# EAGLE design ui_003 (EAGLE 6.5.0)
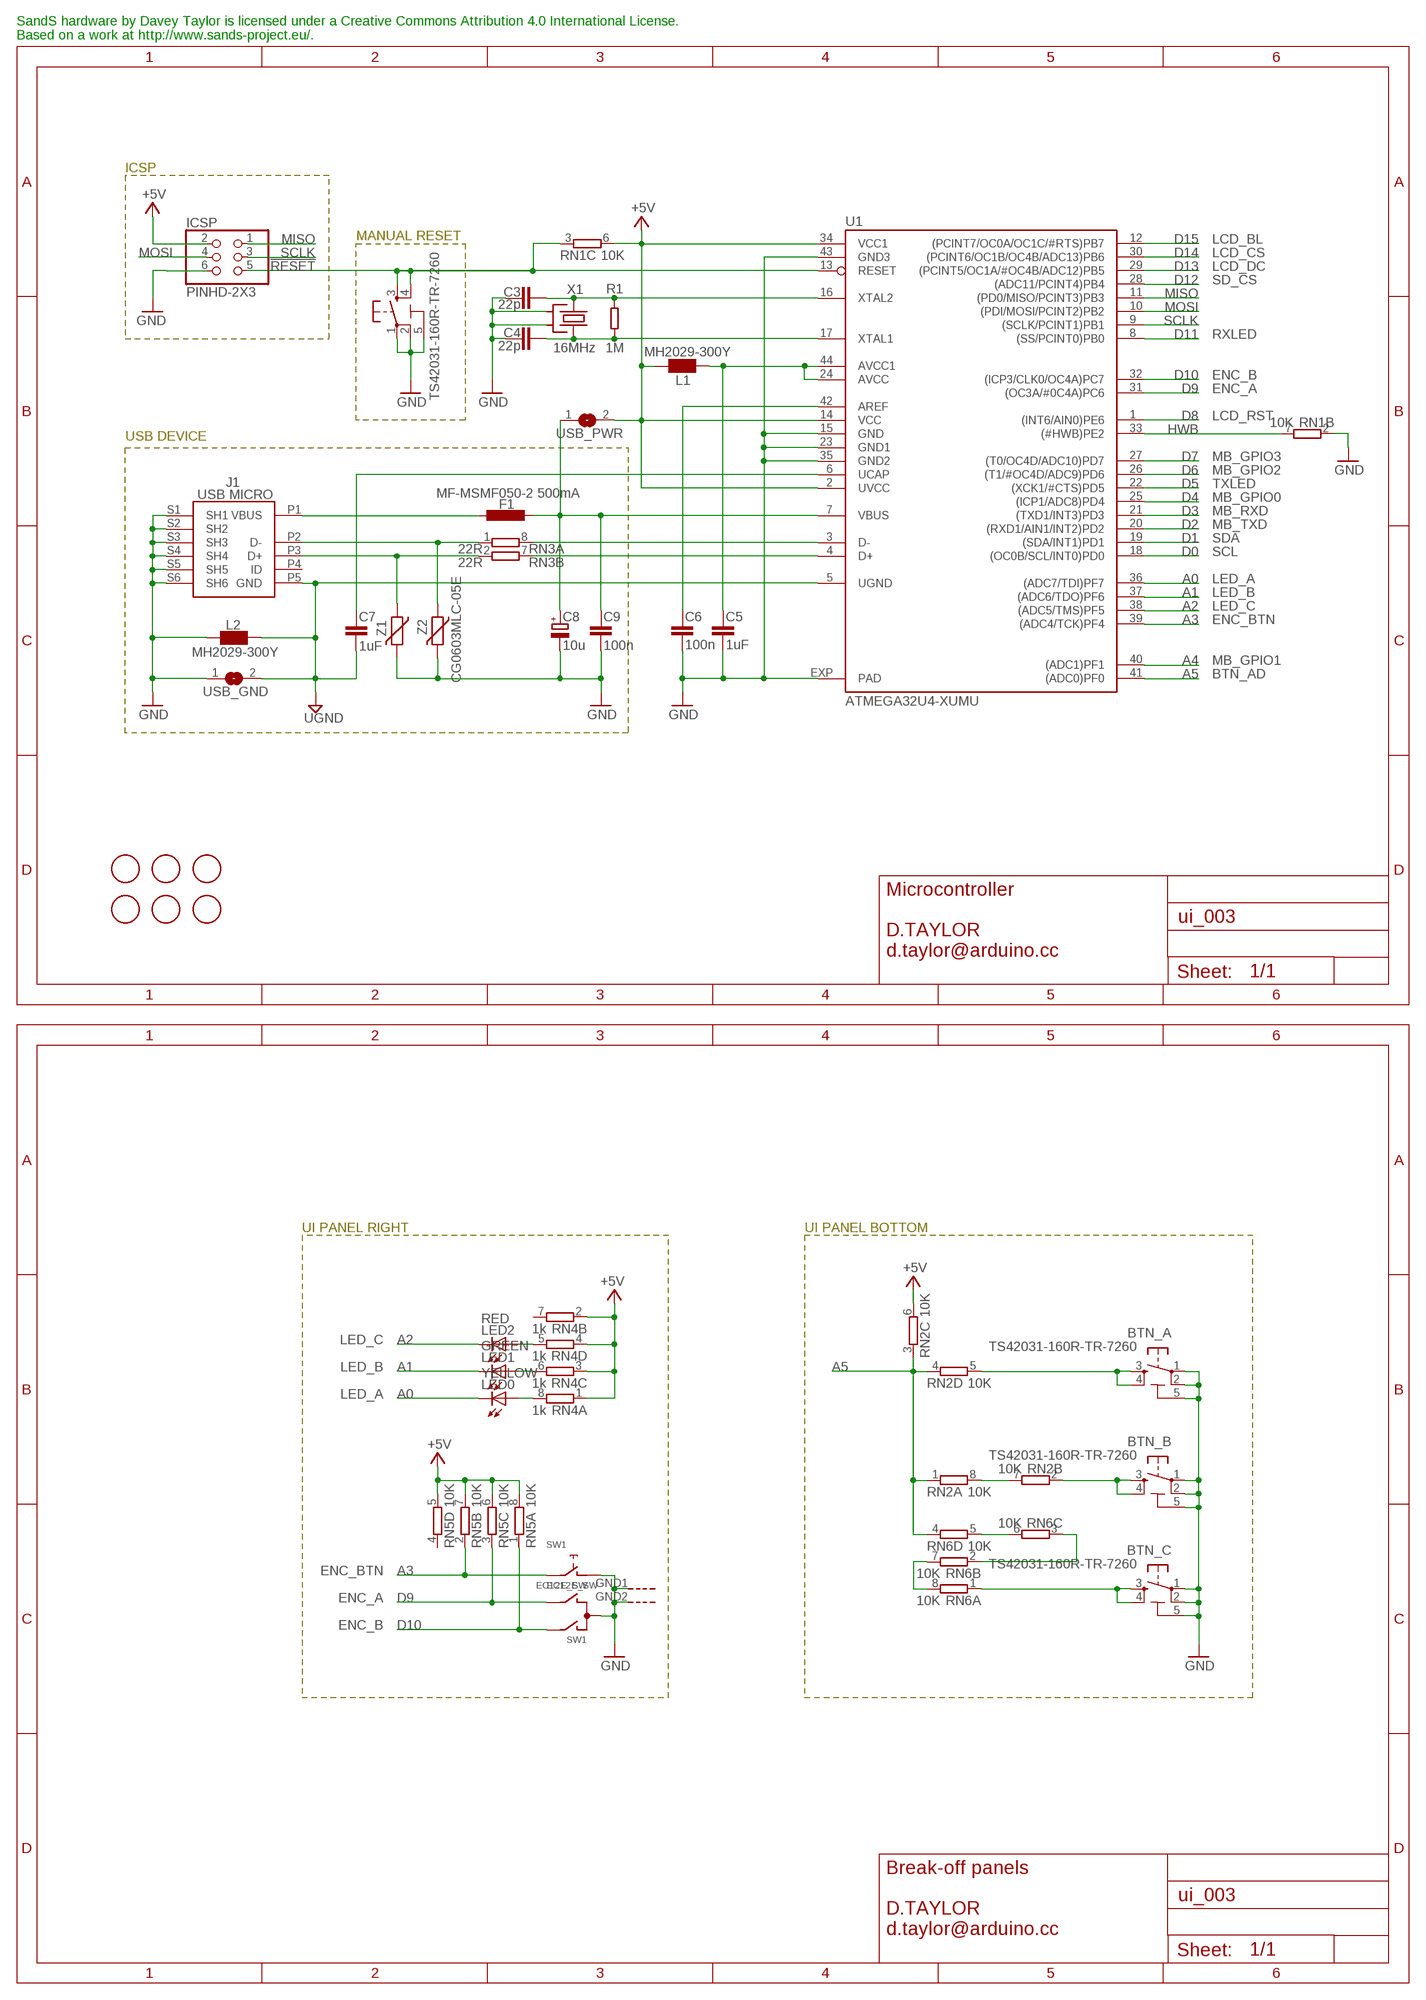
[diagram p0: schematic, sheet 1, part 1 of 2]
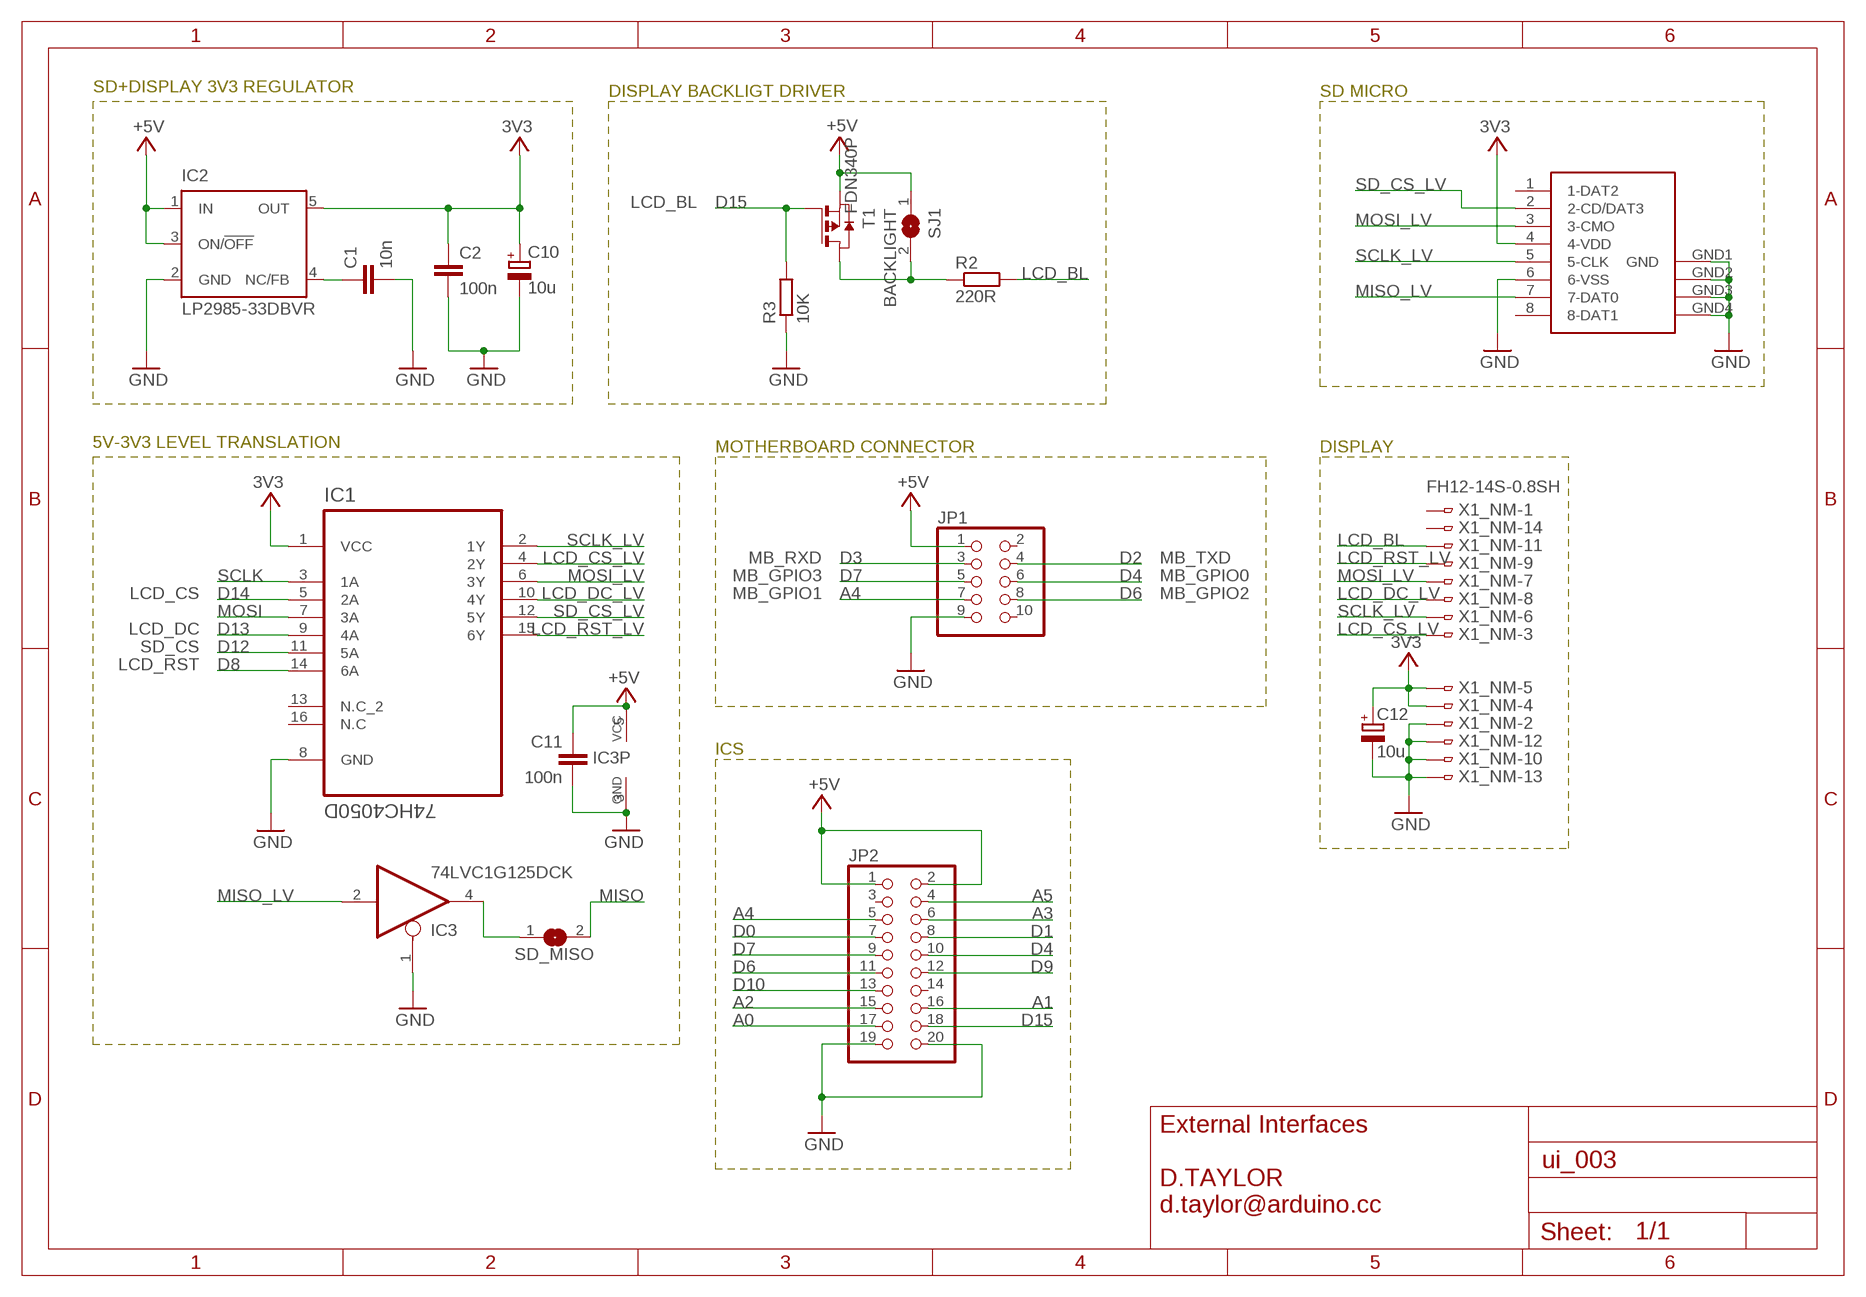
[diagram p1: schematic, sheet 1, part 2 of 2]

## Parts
BTN_A  TS42031-160R-TR-7260  TS42  [TS42]
BTN_B  TS42031-160R-TR-7260  TS42  [TS42]
BTN_C  TS42031-160R-TR-7260  TS42  [TS42]
C1  10n  C-EUC0603  [C0603-ROUND]
C2  100n  C-EUC0603  [C0603-ROUND]
C3  22p  C-EUC0603  [C0603-ROUND]
C4  22p  C-EUC0603  [C0603-ROUND]
C5  1uF  C-EUC0603  [C0603-ROUND]
C6  100n  C-EUC0603  [C0603-ROUND]
C7  1uF  C-EUC0603  [C0603-ROUND]
C8  10u  CPOL-EUSMCB  [SMC_B]
C9  100n  C-EUC0603  [C0603-ROUND]
C10  10u  CPOL-EUSMCB  [SMC_B]
C11  100n  C-EUC0603  [C0603-ROUND]
C12  10u  CPOL-EUSMCB  [SMC_B]
F1  MF-MSMF050-2 500mA  L-EUL1812  [L1812]
FID1  FIDUCIALMOUNT  [FIDUCIA-MOUNT]
FID2  FIDUCIALMOUNT  [FIDUCIA-MOUNT]
FID3  FIDUCIALMOUNT  [FIDUCIA-MOUNT]
FID4  FIDUCIALMOUNT  [FIDUCIA-MOUNT]
FID5  FIDUCIALMOUNT  [FIDUCIA-MOUNT]
FID6  FIDUCIALMOUNT  [FIDUCIA-MOUNT]
IC1  74HC4050D  [SOIC127P600X175-16N]
IC2  LP2985-33DBVR  LP2985-XXDBVR33  [SOT23-DBV]
IC3  74LVC1G125DCK  [SC70-5]
ICSP  PINHD-2X3  [2X03]
J1  USB MICRO  MYCON2_USB-MINI-B  [CON2_USB_MICRO_B_AT]
JP1  PINHD-2X5  [2X05]
JP2  PINHD-2X10  [2X10]
L1  MH2029-300Y  WE-CBF_0805  [0805]
L2  MH2029-300Y  WE-CBF_0805  [0805]
LED0  YELLOW  LEDCHIPLED_0805  [CHIPLED_0805]
LED1  GREEN  LEDCHIPLED_0805  [CHIPLED_0805]
LED2  RED  LEDCHIPLED_0805  [CHIPLED_0805]
R1  1M  R-EU_0603-RND  [R0603-ROUND]
R2  220R  R-EU_0603-RND  [R0603-ROUND]
R3  10K  R-EU_0603-RND  [R0603-ROUND]
RESET  TS42031-160R-TR-7260  TS42  [TS42]
RN1  10K  4R-NCAY16  [CAY16]
RN2  10K  4R-NCAY16  [CAY16]
RN3  22R  4R-NCAY16  [CAY16]
RN4  1k  4R-NCAY16  [CAY16]
RN5  10K  4R-NCAY16  [CAY16]
RN6  10K  4R-NCAY16  [CAY16]
SD_MISO  SJ-NO  [SJ]
SJ1  BACKLIGHT  SJ-NO  [SJ]
SW1  EC12E_SW  [ALPS_EC12E_SW]
T1  FDN340P  [SOT-23]
U1  ATMEGA32U4-XUMU  [QFN44ML7X7]
U2  SDCARD-15TW-8821  [SDCARD-15TW-8821]
USB_GND  SJ-NO  [SJ]
USB_PWR  SJ-NO  [SJ]
X1  16MHz  CRYSTAL2-KX7  [XTAL-3.2-2.5]
X1_NM  FH12-14S-0.8SH  [FH12-14S-0.5SH]
Z1  CG0603MLC-05E  VARISTORCN0603  [CT/CN0603]
Z2  CG0603MLC-05E  VARISTORCN0603  [CT/CN0603]

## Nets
3V3: C2.1 C10.+ C12.+ IC1.1(VCC) IC2.5(OUT) U2.4(4-VDD) X1_NM.4 X1_NM.5
!RESET!: ICSP.5 RESET.3 RESET.4 RN1.3 U1.13(RESET)
+5V [usbvcc]: C11.1 IC2.1(IN) IC2.3(ON/!OFF) IC3.5(VCC) ICSP.2 JP1.1 JP2.1 JP2.2 L1.1 RN1.6 RN2.6 RN4.1 RN4.2 RN4.3 RN4.4 RN5.5 RN5.6 RN5.7 RN5.8 SJ1.1 T1.2(S) U1.2(UVCC) U1.14(VCC) U1.34(VCC1) USB_PWR.2
A0: JP2.17 LED0.C U1.36((ADC7/TDI)PF7)
A1: JP2.16 LED1.C U1.37((ADC6/TDO)PF6)
A2: JP2.15 LED2.C U1.38((ADC5/TMS)PF5)
A3: JP2.6 RN5.2 SW1.E U1.39((ADC4/TCK)PF4)
A4: JP1.7 JP2.5 U1.40((ADC1)PF1)
A5: JP2.4 RN2.1 RN2.3 RN2.4 RN6.4 U1.41((ADC0)PF0)
AREF [aref]: C6.1 U1.42(AREF)
AVCC: C5.1 L1.2 U1.24(AVCC) U1.44(AVCC1)
D0: JP2.7 U1.18((OC0B/SCL/INT0)PD0)
D1: JP2.8 U1.19((SDA/INT1)PD1)
D2: JP1.4 U1.20((RXD1/AIN1/INT2)PD2)
D3: JP1.3 U1.21((TXD1/INT3)PD3)
D4: JP1.6 JP2.10 U1.25((ICP1/ADC8)PD4)
D5: U1.22((XCK1/#CTS)PD5)
D6: JP1.8 JP2.11 U1.26((T1/#OC4D/ADC9)PD6)
D7: JP1.5 JP2.9 U1.27((T0/OC4D/ADC10)PD7)
D8: IC1.14(6A) U1.1((INT6/AIN0)PE6)
D9: JP2.12 RN5.3 SW1.B U1.31((OC3A/#0C4A)PC6)
D10: JP2.13 RN5.1 SW1.A U1.32((ICP3/CLK0/OC4A)PC7)
D11: U1.8((SS/PCINT0)PB0)
D12: IC1.11(5A) U1.28((ADC11/PCINT4)PB4)
D13: IC1.9(4A) U1.29((PCINT5/OC1A/#OC4B/ADC12)PB5)
D14: IC1.5(2A) U1.30((PCINT6/OC1B/OC4B/ADC13)PB6)
D15: JP2.18 R3.2 T1.1(G) U1.12((PCINT7/OC0A/OC1C/#RTS)PB7)
D+: J1.P3(D+) RN3.2 Z1.1
D-: J1.P2(D-) RN3.1 Z2.1
GND [gnd]: BTN_A.1 BTN_A.2 BTN_A.5(5-GND) BTN_B.1 BTN_B.2 BTN_B.5(5-GND) BTN_C.1 BTN_C.2 BTN_C.5(5-GND) C1.2 C2.2 C3.1 C4.2 C5.2 C6.2 C8.- C9.2 C10.- C11.2 C12.- IC1.8(GND) IC2.2(GND) IC3.1(OE) IC3.3(GND) ICSP.6 J1.S1(SH1) J1.S2(SH2) J1.S3(SH3) J1.S4(SH4) J1.S5(SH5) J1.S6(SH6) JP1.9 JP2.19 JP2.20 L2.2 R3.1 RESET.1 RESET.2 RESET.5(5-GND) RN1.2 SW1.C SW1.D SW1.GND1(G) SW1.GND2(G) U1.15(GND) U1.23(GND1) U1.35(GND2) U1.43(GND3) U1.EXP(PAD) U2.6(6-VSS) U2.GND1(GND) U2.GND2(GND1) U2.GND3(GND2) U2.GND4(GND3) USB_GND.1 X1.2(SH1) X1.4(SH2) X1_NM.2 X1_NM.10 X1_NM.12 X1_NM.13 Z1.2 Z2.2
HWB: RN1.7 U1.33((#HWB)PE2)
LCD_BL: R2.2 X1_NM.11
LCD_CS_LV: IC1.4(2Y) X1_NM.3
LCD_DC_LV: IC1.10(4Y) X1_NM.8
LCD_RST_LV: IC1.15(6Y) X1_NM.9
MISO: ICSP.1 SD_MISO.2 U1.11((PD0/MISO/PCINT3)PB3)
MISO_LV: IC3.2(I) U2.7(7-DAT0)
MOSI: IC1.7(3A) ICSP.4 U1.10((PDI/MOSI/PCINT2)PB2)
MOSI_LV: IC1.6(3Y) U2.3(3-CMO) X1_NM.7
N$2: R2.1 SJ1.2 T1.3(D)
N$3: C1.1 IC2.4(NC/FB)
N$4: LED0.A RN4.8
N$5: LED2.A RN4.5
N$6: LED1.A RN4.6
N$7: BTN_A.3 BTN_A.4 RN2.5
N$8: IC3.4(O) SD_MISO.1
N$9: RN2.7 RN2.8
N$10: RN6.5 RN6.6
N$11: BTN_B.3 BTN_B.4 RN2.2
N$12: BTN_C.3 BTN_C.4 RN6.1
N$13: RN6.2 RN6.3
N$14: RN6.7 RN6.8
SCLK: IC1.3(1A) ICSP.3 U1.9((SCLK/PCINT1)PB1)
SCLK_LV: IC1.2(1Y) U2.5(5-CLK) X1_NM.6
SD_CS_LV: IC1.12(5Y) U2.2(2-CD/DAT3)
UCAP: C7.1 U1.6(UCAP)
UGND [gnd]: C7.2 J1.P5(GND) L2.1 U1.5(UGND) USB_GND.2
USB_D+: RN3.7 U1.4(D+)
USB_D-: RN3.8 U1.3(D-)
USB_VCC: C8.+ C9.1 F1.1 U1.7(VBUS) USB_PWR.1
XTAL1: C4.1 R1.1 U1.17(XTAL1) X1.3(X2)
XTAL2: C3.2 R1.2 U1.16(XTAL2) X1.1(X1)
XUSB [usbvcc]: F1.2 J1.P1(VBUS)
Unconnected: IC1.13(N.C_2) IC1.16(N.C) J1.P4(ID) JP1.2 JP1.10 JP2.3 JP2.14 RN1.1 RN1.4 RN1.5 RN1.8 RN3.3 RN3.4 RN3.5 RN3.6 RN4.7 RN5.4 U2.1(1-DAT2) U2.8(8-DAT1) X1_NM.1 X1_NM.14

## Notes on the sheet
- SandS hardware by Davey Taylor is licensed under a Creative Commons Attribution 4.0 International License.
  Based on a work at http://www.sands-project.eu/.
- ICSP
- MANUAL RESET | LCD_BL
- LCD_CS
- LCD_DC
- SD_CS
- RXLED
- ENC_B
- ENC_A
- LCD_RST
- USB DEVICE
- MB_GPIO3
- MB_GPIO2
- TXLED
- MB_GPIO0
- MB_RXD
- MB_TXD
- SDA
- SCL
- LED_A
- LED_B
- LED_C
- ENC_BTN
- MB_GPIO1
- BTN_AD
- Microcontroller
  
  D.TAYLOR
  d.taylor@arduino.cc
- UI PANEL RIGHT | UI PANEL BOTTOM
- LED_C
- LED_B
- LED_A
- ENC_BTN
- ENC_A
- ENC_B
- Break-off panels
  
  D.TAYLOR
  d.taylor@arduino.cc
- SD+DISPLAY 3V3 REGULATOR | DISPLAY BACKLIGT DRIVER | SD MICRO
- LCD_BL
- 5V-3V3 LEVEL TRANSLATION | MOTHERBOARD CONNECTOR | DISPLAY
- MB_RXD | MB_TXD
- MB_GPIO3 | MB_GPIO0
- LCD_CS | MB_GPIO1 | MB_GPIO2
- LCD_DC
- SD_CS
- LCD_RST
- ICS
- External Interfaces
  
  D.TAYLOR
  d.taylor@arduino.cc

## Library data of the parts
BTN_A BTN_B BTN_C RESET = SmartPrj:TS42: TS42 Dongnan Electronics Tact switch VDC 12V - 50mA
C1-C7 C9 C11 = SmartPrj:C-EU: CAPACITOR, European symbol
C8 C12 = rcl:CPOL-EU: POLARIZED CAPACITOR, European symbol
C10 = SmartPrj:CPOL-EU: POLARIZED CAPACITOR, European symbol
F1 = rcl:L-EU: INDUCTOR, European symbol
FID1-FID6 = SmartPrj:FIDUCIALMOUNT
IC1 = SmartPrj:74HC4050D: Hex high-to-low level shifter; MPN: 74HC4050D; OC_FARNELL: 1085272; OC_NEWARK: -; PACKAGE: SOIC-16; SUPPLIER: NXP
IC2 = SmartPrj:LP2985-XXDBVR: ULTRALOW-POWER 50-mA LOW-DROPOUT LINEAR REGULATORS 50-mA Low-Dropout Regulator Source: http://focus.ti.com/lit/ds/symlink/tps77001.pdf
IC3 = 74xx-little-us:74*1G125: Single Bus Buffer Gate with 3-State Output
ICSP = SmartPrj:PINHD-2X3: PIN HEADER
J1 = d_taylor:MYCON2_USB-MINI-B
JP1 = pinhead:PINHD-2X5: PIN HEADER
JP2 = pinhead:PINHD-2X10: PIN HEADER
L1 L2 = wuerth-elektronik:WE-CBF: SMD EMI Suppression Ferrite Beads
LED0 LED1 LED2 = led:LED: LED
R1 = d_taylor:R-EU_: RESISTOR, European symbol
R2 R3 = SmartPrj:R-EU_: RESISTOR, European symbol
RN1-RN6 = resistor-dil:4R-N: Array Chip Resistor Source: RS Component / Phycomp; OC_FARNELL: unknown; OC_NEWARK: unknown
SD_MISO SJ1 USB_GND USB_PWR = d_taylor:SJ?-NO: SMD solder JUMPER
SW1 = switch-alps:EC12E_SW: ALPS rotary Encoder EC12E series with switch; MPN: EC12E2424407; OC_FARNELL: 1520813; OC_NEWARK: 74M1068
T1 = d_taylor:FDN340
U1 = d_taylor:ATMEGA32U4-XU
U2 = st-mod v1.4:SDCARD-15TW-8821: SD Card SDCARD 15TW 8821
X1 = d_taylor:CRYSTAL2: KX7 SMD crystal
X1_NM = con-hirose:FH12-14S-0.8S: 0.5mm Pitch Connectors For FPC/FFC Source: Data sheet; MPN: MC34827; OC_FARNELL: 1324544; OC_NEWARK: 41P0493
Z1 Z2 = varistor:VARISTOR: VARISTOR

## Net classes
0 default: width 0.203 mm, drill 0.406 mm, clearance 0.203 mm
2 gnd: width 0.203 mm, drill 0.406 mm, clearance 0.203 mm
3 usbvcc: width 0.203 mm, drill 0.406 mm, clearance 0.203 mm
4 aref: width 0.203 mm, drill 0.406 mm, clearance 0.203 mm

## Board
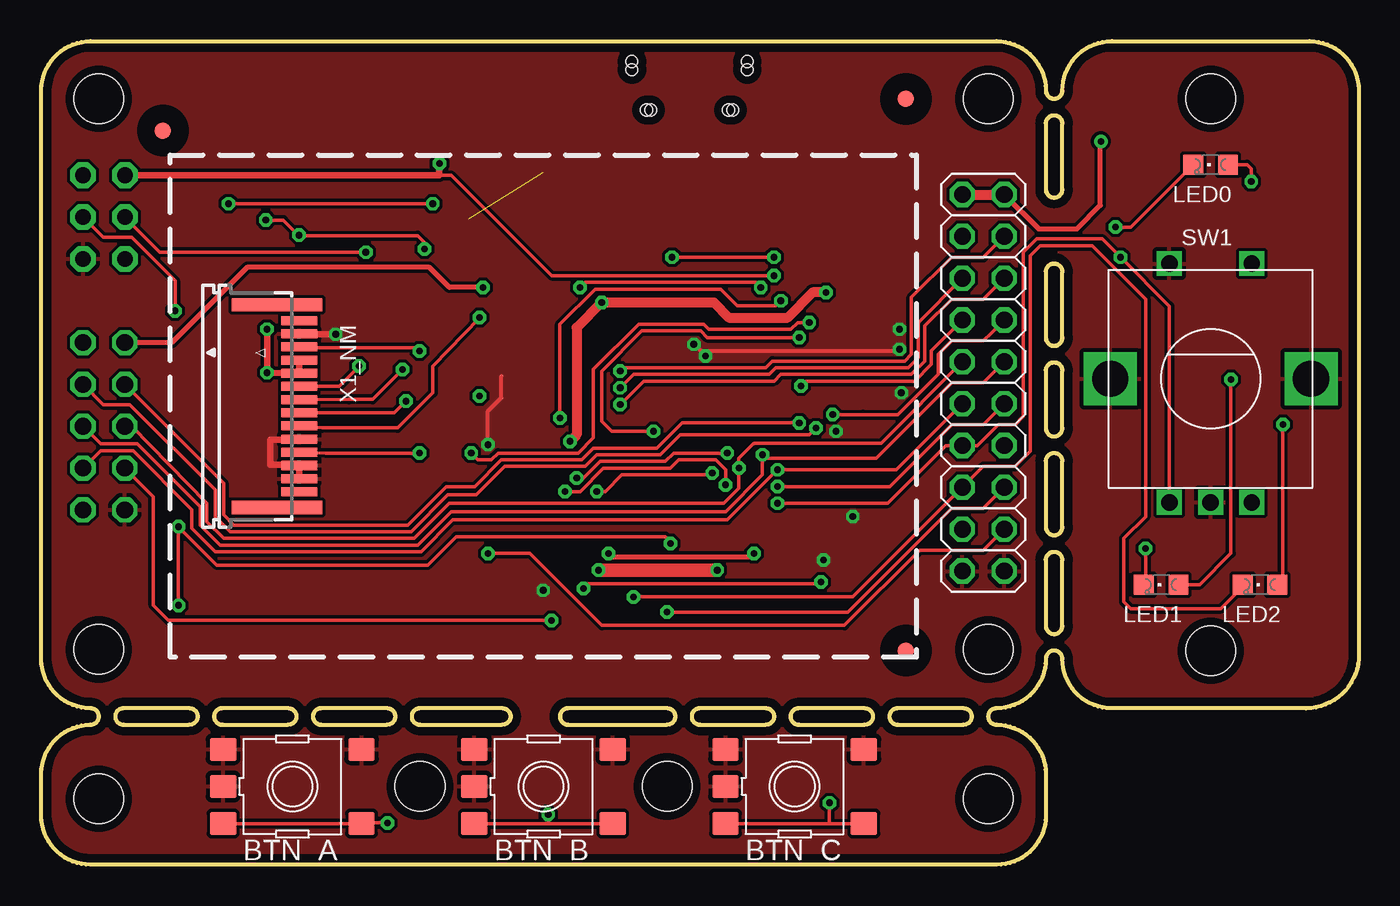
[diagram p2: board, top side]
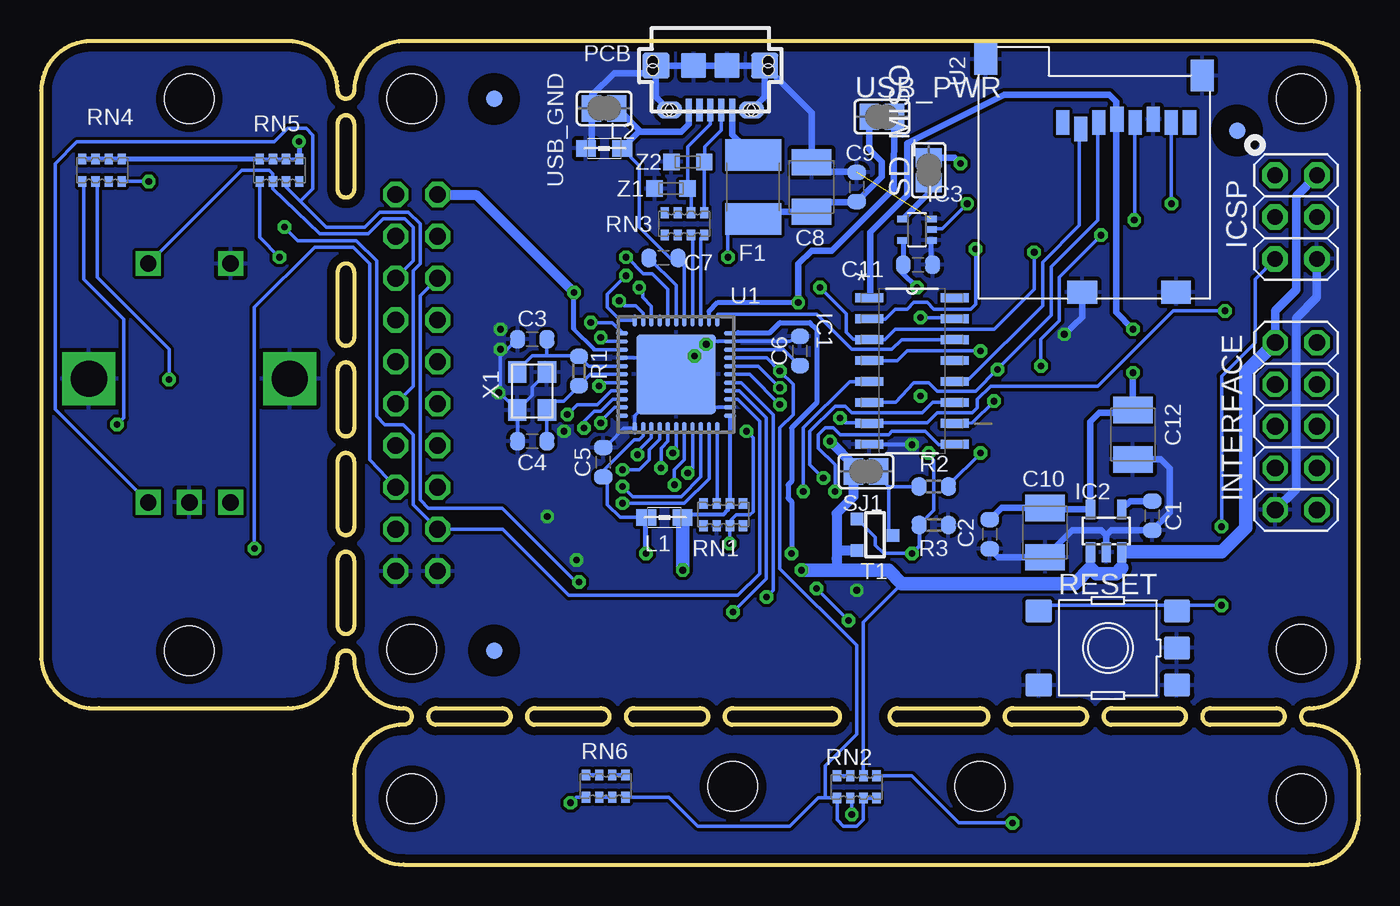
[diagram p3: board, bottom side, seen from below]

Size 80 x 50 mm. Coordinates in mm from the lower left corner, seen from the top.
Outline: 76 segments
Copper layers (1*16): Top 0.035mm / dielectric 1.5mm / Bottom 0.035mm
Design rules "default *": minimum track width 8mil, minimum drill 16mil, track to track 8mil, track to pad 8mil, pad to pad 8mil, via to via 8mil, smd to smd 8mil, copper to edge 20mil, drill to drill 8mil, minimum pad ring 10mil, minimum via ring 8mil, stop-mask expansion 4mil, vias tented up to drill 0mil, thermal gap 10mil
Holes 3 mm at 3.5,46.5 3.5,4 57.5,4 57.5,46.5 3.5,13.07 57.5,13.07 71,46.5 71,13 38,4.75 23,4.75

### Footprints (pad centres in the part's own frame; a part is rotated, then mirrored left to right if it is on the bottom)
TS42 = smd 1.6 x 1.4: 1 -4.2,2.25; 2 4.2,2.25; 3 -4.2,-2.25; 4 4.2,-2.25; 5 -4.2,0
C0603-ROUND = smd 0.898 x 1.1: 1 -0.889,0; 2 0.889,0
SMC_B = smd 1.6 x 2.4: + -1.5,0; - 1.5,0
L1812 = smd 1.9 x 3.4: 1 -1.95,0; 2 1.95,0
FIDUCIA-MOUNT = smd 1.016 x 1.016: P$1 0,0
SOIC127P600X175-16N = smd 1.702 x 0.533: 1 -2.591,4.445; 2 -2.591,3.175; 3 -2.591,1.905; 4 -2.591,0.635; 5 -2.591,-0.635; 6 -2.591,-1.905; 7 -2.591,-3.175; 8 -2.591,-4.445; 9 2.591,-4.445; 10 2.591,-3.175; 11 2.591,-1.905; 12 2.591,-0.635; 13 2.591,0.635; 14 2.591,1.905; 15 2.591,3.175; 16 2.591,4.445
SOT23-DBV = smd 0.55 x 1.2: 1 -0.95,-1.3; 2 0,-1.3; 3 0.95,-1.3; 4 0.95,1.3; 5 -0.95,1.3
SC70-5 = smd 0.4 x 0.7: 1 -0.65,-0.85; 2 0,-0.85; 3 0.65,-0.85; 4 0.65,0.85; 5 -0.65,0.85
2X03 = drill 0.95 pad 1.55 octagon: 1 -2.54,-1.27; 2 -2.54,1.27; 3 0,-1.27; 4 0,1.27; 5 2.54,-1.27; 6 2.54,1.27
CON2_USB_MICRO_B_AT = smd 0.406 x 1.346: P1 -1.321,2.692; P2 -0.66,2.692; P3 0,2.692; P4 0.66,2.692; P5 1.321,2.692 | smd 1.651 x 1.549: S1 -3.302,0; S2 3.302,0 | smd 1.524 x 1.016: S3 -2.489,2.692; S4 2.489,2.692 | smd 1.524 x 1.524: S5 -1.016,0; S6 1.016,0 | hole 0.7: -3.505,0.254; -3.505,-0.254; 3.505,0.254; 3.505,-0.254; -2.616,2.692; -2.362,2.692; 2.362,2.692; 2.616,2.692
2X05 = drill 1.016 octagon: 1 -5.08,-1.27; 2 -5.08,1.27; 3 -2.54,-1.27; 4 -2.54,1.27; 5 0,-1.27; 6 0,1.27; 7 2.54,-1.27; 8 2.54,1.27; 9 5.08,-1.27; 10 5.08,1.27
2X10 = drill 1.016 octagon: 1 -11.43,-1.27; 2 -11.43,1.27; 3 -8.89,-1.27; 4 -8.89,1.27; 5 -6.35,-1.27; 6 -6.35,1.27; 7 -3.81,-1.27; 8 -3.81,1.27; 9 -1.27,-1.27; 10 -1.27,1.27; 11 1.27,-1.27; 12 1.27,1.27; 13 3.81,-1.27; 14 3.81,1.27; 15 6.35,-1.27; 16 6.35,1.27; 17 8.89,-1.27; 18 8.89,1.27; 19 11.43,-1.27; 20 11.43,1.27
0805 = smd 1.2 x 1: 1 -1.1,0; 2 1.1,0
CHIPLED_0805 = smd 1.2 x 1.2: A 0,-1.05; C 0,1.05
R0603-ROUND = smd 0.898 x 1.1: 1 -0.889,0; 2 0.889,0
CAY16 = smd 0.5 x 0.65: 1 -1.2,-0.675; 2 -0.4,-0.675; 3 0.4,-0.675; 4 1.2,-0.675; 5 1.2,0.675; 6 0.4,0.675; 7 -0.4,0.675; 8 -1.2,0.675
SJ = smd 1.168 x 1.6: 1 -0.762,0; 2 0.762,0
ALPS_EC12E_SW = drill 1 square: A -2.5,-7.5; B 2.5,-7.5; C 0,-7.5; D -2.5,7; E 2.5,7 | drill 2.2 square: GND1 -6.1,0; GND2 6.1,0
SOT-23 = smd 0.762 x 0.762: 1 -0.979,-1.101; 2 0.94,-1.101; 3 0.025,1.067
QFN44ML7X7 = smd 0.75 x 0.275: 1 -3.275,2.5; 2 -3.275,2; 3 -3.275,1.5; 4 -3.275,1; 5 -3.275,0.5; 6 -3.275,0; 7 -3.275,-0.5; 8 -3.275,-1; 9 -3.275,-1.5; 10 -3.275,-2; 11 -3.275,-2.5; 23 3.275,-2.5; 24 3.275,-2; 25 3.275,-1.5; 26 3.275,-1; 27 3.275,-0.5; 28 3.275,0; 29 3.275,0.5; 30 3.275,1; 31 3.275,1.5; 32 3.275,2; 33 3.275,2.5 | smd 0.275 x 0.75: 12 -2.5,-3.275; 13 -2,-3.275; 14 -1.5,-3.275; 15 -1,-3.275; 16 -0.5,-3.275; 17 0,-3.275; 18 0.5,-3.275; 19 1,-3.275; 20 1.5,-3.275; 21 2,-3.275; 22 2.5,-3.275; 34 2.5,3.275; 35 2,3.275; 36 1.5,3.275; 37 1,3.275; 38 0.5,3.275; 39 0,3.275; 40 -0.5,3.275; 41 -1,3.275; 42 -1.5,3.275; 43 -2,3.275; 44 -2.5,3.275 | smd 4.826 x 4.826: EXP 0,0
SDCARD-15TW-8821 = smd 0.8 x 1.5: 1 0,0; 2 1.1,-0.4; 3 2.2,0; 4 3.3,0.2; 5 4.4,0; 6 5.5,0.2; 7 6.6,0; 8 7.7,0 | smd 1.4 x 1.9: GND1 -4.66,3.85; GND2 8.49,2.85 | smd 1.8 x 1.4: GND3 1.19,-10.3; GND4 6.89,-10.3
XTAL-3.2-2.5 = smd 1.3 x 1.1: 1 -1.15,-0.9; 2 1.15,-0.9; 3 1.15,0.9; 4 -1.15,0.9
FH12-14S-0.5SH = smd 0.55 x 2.2: 1 -5.2,3.25; 2 -4.4,3.25; 3 -3.6,3.25; 4 -2.8,3.25; 5 -2,3.25; 6 -1.2,3.25; 7 -0.4,3.25; 8 0.4,3.25; 9 1.2,3.25; 10 2,3.25; 11 2.8,3.25; 12 3.6,3.25; 13 4.4,3.25; 14 5.2,3.25 | smd 0.8 x 5.5: P1 -6.15,1.9; P2 6.15,1.9
CT/CN0603 = smd 1 x 1: 1 -1,0; 2 1,0

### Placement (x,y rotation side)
BTN_A  15.25,4.75 0 top
BTN_B  30.5,4.75 0 top
BTN_C  45.75,4.75 0 top
C1  12.55,21.18 270 bottom
C2  22.4,20.07 270 bottom
C3  50.19,31.9 0 bottom
C4  50.19,25.7 180 bottom
C5  45.87,24.43 90 bottom
C6  33.93,31.19 90 bottom
C7  42.21,36.83 0 bottom
C8  33.22,41.15 90 bottom
C9  30.48,41.15 90 bottom
C10  19.05,20.17 270 bottom
C11  26.77,36.42 0 bottom
C12  13.72,26.11 270 bottom
F1  36.78,41.15 90 bottom
FID1  52.5,13 0 bottom
FID2  7.38,44.57 0 bottom
FID3  52.5,46.5 0 bottom
FID4  7.38,44.57 0 top
FID5  52.5,46.5 0 top
FID6  52.5,13 0 top
IC1  27.13,29.97 0 bottom
IC2  15.34,20.27 0 bottom
IC3  26.82,38.56 90 bottom
ICSP  3.81,39.32 270 bottom
J1  39.37,48.51 180 bottom
JP1  3.81,26.62 270 bottom
JP2  57.2,29.26 270 top
L1  42.16,21.08 180 bottom
L2  45.82,43.48 180 bottom
LED0  71,42.5 90 top
LED1  68,17 90 top
LED2  74,17 90 top
R1  47.35,29.97 90 bottom
R2  25.81,22.96 0 bottom
R3  25.81,20.62 180 bottom
RESET  15.24,13.16 180 bottom
RN1  38.58,21.26 0 bottom
RN2  30.48,4.72 0 bottom
RN3  40.94,38.91 180 bottom
RN4  76.3,42.16 180 bottom
RN5  65.53,42.16 0 bottom
RN6  45.72,4.78 0 bottom
SD_MISO  26.11,42.16 90 bottom
SJ1  29.92,23.88 0 bottom
SW1  71,29.5 0 top
T1  29.36,20.02 270 bottom
U1  41.45,29.77 270 bottom
U2  17.98,45.06 0 bottom
USB_GND  45.82,45.92 0 bottom
USB_PWR  28.96,45.42 0 bottom
X1  50.19,28.75 270 bottom
X1_NM  12.42,27.84 270 top
Z1  41.76,41.05 180 bottom
Z2  40.74,42.67 180 bottom

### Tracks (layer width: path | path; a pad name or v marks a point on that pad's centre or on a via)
3V3  (via drill 0.41)
  Top 0.406: v13.72,32.51 v13.72,29.87 15.61,29.84 X1_NM.5 X1_NM.4
  Bottom 0.203: 14.73,44.91 U2.4 14.73,45.31
  Bottom 0.406: v13.72,32.51 14.73,33.53 14.73,44.91 | IC1.1 29.69,34.42 29.67,34.44 29.67,38.41 27.43,40.64 27.43,43.79 21.54,46.74 15.14,46.74 14.73,46.33 14.73,45.31 | C2.1 21.69,21.67 C10.+ 18.95,21.57 IC2.5 16.29,26.89 15.75,27.43 13.89,27.43 C12.+ v13.72,29.87
!RESET!  (via drill 0.41)
  Top 0.203: v8.33,15.75 v8.33,20.52 10.67,18.19 23.47,18.19 25.2,19.91 37.9,19.91 v38.2,19.51 | v37.19,26.31 34.65,26.31 34.04,26.92 34.04,29.97 36.47,32.41 40.03,32.41 40.44,32 v46.02,32
  Bottom 0.203: ICSP.5 6.3,35.56 6.3,31.7 8.33,29.67 v8.33,20.52 | RESET.3 10.69,15.75 v8.33,15.75 18.93,15.75 RESET.4 | v38.2,19.51 38.2,20.42 RN1.3 38.1,20.77 38.1,20.93 37.8,21.23 36.98,21.23 36.78,21.44 36.78,25.91 v37.19,26.31 | v46.02,32 45.79,31.77 U1.13
+5V  (via drill 0.41)
  Top 0.305: v26.82,35.05 24.79,35.05 23.57,36.27 12.5,36.27 7.92,31.7 JP1.1 | JP2.2 60.55,38.61 62.89,38.61 64.31,40.03 64.31,43.89 v64.34,43.92
  Top 0.61: v32.11,25.7 32.51,26.11 32.51,32.61 v34.04,34.14 40.84,34.14 41.76,33.22 45.31,33.22 46.84,34.75 v47.65,34.75 | JP2.1 JP2.2
  Top 0.813: v41.05,17.88 v33.83,17.88
  Bottom 0.203: 41.05,21.26 L1.1 | 27.67,36.44 C11.1 27.74,36.6 | 27.74,17.07 30.07,14.73 30.07,5.49 RN2.6 | 38.28,21.66 38.28,21.86 RN1.6 38.18,22.04 | U1.14 46.41,31.27 46.43,31.29 | RN5.8 RN5.7 RN5.6 RN5.5
  Bottom 0.254: 41.05,21.26 38.58,21.26 38.3,21.54 38.28,21.66 | U1.2 39.45,33.6 | 38.18,22.04 U1.34 | 46.43,31.29 47.65,32.51 | 30.73,18.03 30.89,17.88
  Bottom 0.305: IC3.5 27.67,36.44 | 27.74,36.6 27.74,35.97 v26.82,35.05 | 3.86,40.54 3.81,40.59 | 39.45,33.6 38.91,34.14 v34.04,34.14 | 30.68,24.28 SJ1.1 | 47.65,32.51 v47.65,34.75 | L1.1 41.06,20.85 41.05,20.83 | RN4.4 RN4.3 RN4.2 RN4.1 RN5.8 | v64.34,43.92 RN5.5
  Bottom 0.406: IC2.3 14.39,18.02 | IC2.1 16.29,18.02 | 17.24,17.07 17.27,17.07 | USB_PWR.2 28.25,41.05 32,37.29 33.22,37.29 34.04,36.47 v34.04,34.14
  Bottom 0.508: IC2.3 14.36,18.97 14.22,19 | JP1.1 5.08,33.63 3.81,34.9 3.81,40.59 ICSP.2
  Bottom 0.61: v32.11,25.7 30.68,24.28 | v47.65,34.75 53.54,40.64 55.88,40.64 JP2.1 | SJ1.1 30.68,22.35 31.7,21.34 31.7,18.59 | 31.7,18.59 31.7,17.88 | T1.2 31.67,19.07 31.7,18.59
  Bottom 0.813: 14.39,18.02 14.73,17.68 15.95,17.68 16.29,18.02 17.24,17.07 | 14.22,19 8.33,19 6.86,20.47 6.86,29.92 JP1.1 | 17.27,17.07 27.74,17.07 28.55,17.88 30.89,17.88 31.7,17.88 v33.83,17.88 | 41.05,20.83 v41.05,17.88
A0  (via drill 0.41)
  Top 0.203: LED0.C 66.16,38.71 v65.23,38.71
  Bottom 0.203: U1.36 37.72,28.27 36.37,26.92 36.37,17.68 37.69,16.36 47.95,16.36 51.97,20.37 JP2.17 57.4,21.84 57.4,26.11 58.01,26.72 59.13,26.72 59.64,27.23 59.64,36.68 60.86,37.9 64.41,37.9 v65.23,38.71
A1  (via drill 0.41)
  Top 0.203: v38,15.34 48.97,15.34 55.27,21.64 57.2,21.64 JP2.16 | v67.06,19.2 67.06,17.11 LED1.C
  Bottom 0.203: U1.37 37.61,28.77 35.97,27.13 35.97,17.37 v38,15.34 | JP2.16 60.05,24.59 60.05,36.47 61.06,37.49 63.4,37.49 67.06,33.83 v67.06,19.2
A2  (via drill 0.41)
  Top 0.203: v35.97,16.26 49.28,16.26 JP2.15 57.2,24.18 59.13,24.18 60.05,25.09 60.05,36.98 60.66,37.59 63.8,37.59 67.06,34.34 67.06,21.13 65.73,19.81 65.73,15.95 66.14,15.54 71.63,15.54 72.95,16.87 LED2.C
  Bottom 0.203: U1.38 37.5,29.27 35.56,27.33 35.56,16.66 v35.97,16.26
A3  (via drill 0.41)
  Top 0.203: v35.15,27.94 36.58,29.36 44.5,29.36 44.91,29.77 52.83,29.77 53.65,30.58 53.65,32.72 55.27,34.34 57.2,34.34 JP2.6
  Bottom 0.203: U1.39 36.98,29.77 v35.15,27.94 | JP2.6 57.4,36.68 57.4,38.71 57.91,39.22 59.23,39.22 60.15,38.3 63.09,38.3 65.94,41.05 RN5.2 65.94,41.8 65.94,41.96 66.14,42.16 67.84,42.16 SW1.E
A4  (via drill 0.41)
  Top 0.203: v35.15,28.96 35.97,29.77 44.2,29.77 44.6,30.18 52.63,30.18 53.24,30.79 53.24,32.92 JP2.5 | v47.35,17.17 47.24,17.07 33.22,17.07 v32.92,16.76 | v30.99,14.83 7.72,14.83 6.81,15.75 6.81,22.35 JP1.7
  Bottom 0.203: U1.40 36.47,30.27 v35.15,28.96 | JP2.5 57,34.54 57,22.15 56.49,21.64 52.02,21.64 47.55,17.17 v47.35,17.17 | v32.92,16.76 v30.99,14.83
A5  (via drill 0.41)
  Top 0.203: v35.15,29.97 35.36,30.18 43.99,30.18 44.4,30.58 52.43,30.58 52.83,30.99 52.83,34.44 55.27,36.88 57.2,36.88 JP2.4
  Bottom 0.203: RN6.4 41.9,4.1 40.13,2.34 34.54,2.34 32.82,4.06 32.41,4.06 | 32.41,4.06 31.7,4.06 RN2.1 31.68,2.72 31.29,2.34 30.48,2.34 30.07,2.74 RN2.3 30.06,4.03 29.26,4.03 RN2.4 | U1.41 35.95,30.77 v35.15,29.97 34.34,29.16 34.34,27.33 35.15,26.52 35.15,17.98 30.48,13.31 30.48,7.92 32.41,5.99 32.41,4.06
AREF
  Bottom 0.203: U1.42 34.9,31.27 C6.1
AVCC  (via drill 0.41)
  Top 0.305: v34.44,18.9 34.65,18.69 43.08,18.69 v43.28,18.9
  Bottom 0.203: 43.45,21.08 L1.2 44.86,21.08 45.62,21.84 45.62,23.27 45.87,23.52 C5.1 45.82,23.98 43.99,25.81 43.69,25.81 43.46,26.04 U1.24
  Bottom 0.254: U1.44 37.73,32.27 37.69,32.31
  Bottom 0.305: 37.69,32.31 35.76,32.31 35.15,32.92 33.33,32.92 32.92,32.51 32.92,28.04 34.44,26.52 34.44,23.27 34.65,23.06 34.65,22.25 34.44,22.05 v34.44,18.9 | v43.28,18.9 43.28,21.06 L1.2
D0  (via drill 0.41)
  Top 0.203: v46.13,29.06 46.43,29.36 53.03,29.36 54.05,30.38 54.05,31.19 JP2.7
  Bottom 0.203: U1.18 45.91,29.27 v46.13,29.06
D1  (via drill 0.41)
  Top 0.203: v48.06,27.33 49.89,27.33 52.02,27.33 54.46,29.77 54.46,30.99 55.27,31.8 57.2,31.8 57.71,32.31 JP2.8
  Bottom 0.203: U1.19 45.4,28.77 46.23,27.94 47.45,27.94 v48.06,27.33
D2  (via drill 0.41)
  Top 0.203: JP1.4 3.76,27.94 5.38,27.94 10.57,22.76 10.57,21.13 11.48,20.22 22.45,20.22 24.69,22.45 26.42,22.45 28.14,24.18 33.02,24.18 33.73,24.89 37.59,24.89 38.81,26.11 46.63,26.11 v47.04,26.52
  Bottom 0.203: v47.04,26.52 47.04,26.92 46.43,27.53 46.02,27.53 45.29,28.27 U1.20
D3  (via drill 0.41)
  Top 0.203: v46.02,26.82 38.91,26.82 37.39,25.3 33.53,25.3 32.82,24.59 27.94,24.59 26.31,22.96 24.59,22.96 22.25,20.62 11.68,20.62 11.07,21.23 11.07,23.16 JP1.3
  Bottom 0.203: U1.21 45.18,27.77 46.02,26.92 v46.02,26.82
D4  (via drill 0.41)
  Top 0.203: JP1.6 3.61,25.55 5.84,25.55 9.65,21.74 9.65,20.62 10.87,19.41 22.86,19.41 24.89,21.44 41.55,21.44 43.79,23.67 v43.79,24.89 43.92,24.76 arc45 44.1,24.69 50.7,24.69 55.27,29.26 57.2,29.26 JP2.10
  Bottom 0.203: U1.25 42.95,25.93 43.79,25.09 v43.79,24.89
D6  (via drill 0.41)
  Top 0.203: JP1.8 3.61,25.15 5.59,25.15 9.14,21.54 9.14,20.42 10.57,19 23.06,19 24.99,20.93 41.66,20.93 v44.7,23.98 51.92,23.98 JP2.11
  Bottom 0.203: U1.26 42.45,25.82 43.08,25.2 43.08,24.59 43.69,23.98 v44.7,23.98
D7  (via drill 0.41)
  Top 0.203: JP1.5 5.49,26.62 10.06,21.95 10.06,20.83 11.07,19.81 22.66,19.81 24.79,21.95 41.45,21.95 42.37,22.86 v42.37,24.08 42.37,24.69 43.21,25.53 arc-45 43.39,25.6 51,25.6 JP2.9
  Bottom 0.203: U1.27 41.95,25.71 42.37,25.3 v42.37,24.08
D8
  Bottom 0.203: IC1.14 27.76,31.88 28.35,31.29 30.79,31.29 32.92,33.43 38.91,33.43 U1.1
D9  (via drill 0.41)
  Top 0.203: v44.7,22.96 51.51,22.96 55.27,26.72 57.2,26.72 JP2.12
  Bottom 0.203: U1.31 39.95,23.55 41.15,22.35 44.09,22.35 v44.7,22.96 | JP2.12 57.4,29.06 57.4,36.07 57,36.47 57,38.91 57.71,39.62 59.44,39.62 60.35,38.71 62.69,38.71 64.26,40.28 | 64.26,40.28 65.12,41.14 RN5.3 | SW1.B 79.15,27.65 79.15,42.57 77.83,43.89 65.84,43.89 65.02,44.7 63.91,44.7 63.5,44.3 63.5,41.05 64.26,40.28
D10  (via drill 0.41)
  Top 0.203: v44.7,21.95 51.41,21.95 54.91,25.45 JP2.13 56.84,25.45 58.12,26.72 59.13,26.72 59.64,27.23 59.64,37.19 60.45,38 64.41,38 v65.53,36.88 68.5,33.91 SW1.A
  Bottom 0.203: U1.32 39.45,23.44 40.95,21.95 v44.7,21.95 44.91,21.95 | v65.53,36.88 66.73,38.08 RN5.1
D12  (via drill 0.41)
  Top 0.203: v41.66,24.99 38.41,24.99 37.9,24.49 33.93,24.49 32.92,23.47 v32.51,23.47
  Bottom 0.203: IC1.11 25.88,28.07 26.52,27.43 30.79,27.43 31.19,27.84 31.8,27.84 33.33,26.31 33.33,24.28 v32.51,23.47 | U1.28 41.45,25.2 v41.66,24.99
D13  (via drill 0.41)
  Top 0.203: v41.55,23.06 41.55,23.98 40.95,24.59 38.71,24.59 38.2,24.08 34.14,24.08 32.72,22.66 v31.8,22.66
  Bottom 0.203: U1.29 40.95,24.59 41.55,23.98 v41.55,23.06 | v31.8,22.66 31.8,24.28 32.82,25.3 32.82,26.11 32.41,26.52 31.9,26.52 31.5,26.11 28.55,26.11 28.35,26.31 26.31,26.31 25.5,25.5 24.56,25.5 IC1.9
D14  (via drill 0.41)
  Top 0.203: v33.73,22.66 34.24,22.66 35.26,23.67 40.64,23.67 v40.74,23.77
  Bottom 0.203: v40.74,23.77 40.45,24.06 U1.30 | v33.73,22.66 33.73,26.52 30.91,29.34 IC1.5
D15  (via drill 0.41)
  Top 0.203: v26.11,24.99 26.52,24.59 27.33,24.59 27.74,24.99 32.61,24.99 33.53,25.91 33.53,30.07 36.27,32.82 40.23,32.82 40.54,32.51 45.52,32.51 45.92,32.92 v46.63,32.92 | v27.13,18.9 29.67,18.9 34.04,14.53 48.77,14.53 53.34,19.1 57.2,19.1 JP2.18
  Bottom 0.203: R3.2 25.81,21.51 25.81,24.49 v26.11,24.99 | U1.12 44.73,32.33 45.31,32.92 v46.63,32.92 | v27.13,18.9 28.85,18.9 29.36,19.41 29.36,19.89 T1.1
  Bottom 0.254: R3.2 26.7,19.33 v27.13,18.9
D+
  Bottom 0.203: J1.P3 39.37,44.96 40.74,43.59 40.74,41.06 | RN3.2 40.55,40.83
  Bottom 0.305: 40.74,41.06 Z1.1 40.55,40.83
D-
  Bottom 0.203: J1.P2 38.71,44.6 39.73,43.59 39.73,42.69 | Z2.1 39.74,39.69
  Bottom 0.305: 39.73,42.69 Z2.1 | 39.74,39.69 RN3.1
GND  (via drill 0.41)  (1 unrouted)
  Top 0.254: 40.03,31.19 52.02,31.19 v52.12,31.29 | v40.34,30.89 40.03,31.19 | 40.03,31.19 v39.62,31.6 | v27.13,25.5 27.13,27.53 27.94,28.35 27.94,29.67
  Top 0.406: X1_NM.13 X1_NM.12 14.94,24.28 13.92,24.28 13.92,25.81 14.83,25.81 15.37,25.84 X1_NM.10 | v17.88,32.21 16.2,32.21 X1_NM.2
  Bottom 0.203: U1.EXP v40.34,30.89 v39.62,31.6 39.45,31.77 U1.43 34.55,31.77 C6.2 | U1.35 39.45,27.77 U1.EXP | U1.EXP 43.95,27.27 U1.23 44.63,26.49 45.52,25.6 C5.2 | U1.15 42.45,30.77 U1.EXP | X1.4 50.19,29 50.19,28.5 X1.2 | C11.2 25.97,36.51 | C4.2 X1.2 | C3.1 51.1,31.9 52.02,30.99 52.12,30.89 52.12,28.63 X1.2
  Bottom 0.254: v52.12,31.29 52.12,30.99 52.02,30.99 | IC1.8 27.15,25.53 v27.13,25.5
  Bottom 0.305: 25.97,36.51 IC3.1
  Bottom 0.406: J1.S2 J1.S6 J1.S5 J1.S1 | J1.S1 36.07,46.63 J1.S3 | J1.S2 42.67,46.63 J1.S4 | J1.S2 43.13,48.06 45.21,48.06 46.53,46.74 USB_GND.1 46.58,43.82 L2.2 | J1.S1 33.22,45.67 C8.- 32.64,42.06 30.79,42.06 30.76,42.04 C9.2 | 15.34,20.02 15.04,20.32 12.9,20.32 C1.2 11.48,21.36 11.48,24.08 12.01,24.61 C12.- | 15.34,20.02 IC2.2 | C2.2 21.89,18.67 C10.- 17.4,20.32 15.65,20.32 15.34,20.02 | U2.GND3 16.79,33.25 v17.88,32.21
  Bottom 0.508: JP1.9 3.81,22.81 3.81,33.17 2.54,34.44 ICSP.6
  other vias: 47.5,18.5 30.48,16.66 52.12,32.51 48.26,26.31 52.22,28.65 49.28,21.13
  pour Top: 80,50 0,50 0,0 61,0 61,9.5 80,9.5
  pour Bottom: 80,50 0,50 0,0 61,0 61,9.5 80,9.5
HWB
  Bottom 0.203: U1.33 38.95,22.07 RN1.7
LCD_BL  (via drill 0.41)
  Top 0.203: v22.96,24.99 17.29,24.99 X1_NM.11
  Bottom 0.203: v22.96,24.99 24.92,23.04 R2.2
LCD_CS_LV  (via drill 0.41)
  Top 0.203: X1_NM.3 16.49,31.39 22.76,31.39 v22.96,31.19
  Bottom 0.203: IC1.4 28.02,30.61 27.43,31.19 v22.96,31.19
LCD_DC_LV  (via drill 0.41)
  Top 0.203: v22.15,28.14 21.44,27.44 X1_NM.8
  Bottom 0.203: IC1.10 24,26.8 23.47,26.82 v22.15,28.14
LCD_RST_LV  (via drill 0.41)
  Top 0.203: v26.62,33.22 23.77,30.28 23.77,28.65 21.64,26.52 17.06,26.52 X1_NM.9
  Bottom 0.203: IC1.15 24.41,33.15 24.38,33.12 23.88,33.22 v26.62,33.22
MISO  (via drill 0.41)
  Top 0.203: 24.18,41.86 24.89,41.86 30.99,35.76 v44.5,35.76
  Top 0.406: v24.18,42.57 24.18,41.86 ICSP.1
  Bottom 0.203: v44.5,35.76 45.62,34.65 45.62,33.83 44.83,33.04 U1.11
  Bottom 0.406: SD_MISO.2 24.54,42.93 v24.18,42.57
MISO_LV  (via drill 0.41)
  Top 0.203: v23.77,40.13 v11.38,40.13
  Bottom 0.203: v23.77,40.13 25.3,38.61 25.92,38.61 IC3.2 | v11.38,40.13 U2.7
MOSI  (via drill 0.41)
  Top 0.203: ICSP.4 3.76,38.1 5.49,38.1 8.13,35.46 v8.13,33.63 | v44.91,34.24 44.6,33.93 42.27,33.93 41.25,34.95 33.63,34.95 31.5,32.82 v31.5,27.13
  Bottom 0.203: v8.13,33.63 11.28,33.63 15.85,29.06 22.35,29.06 23.16,28.25 23.16,27.74 23.47,27.43 25.6,27.43 26.21,26.82 29.46,26.82 29.49,26.8 IC1.7 29.74,26.82 31.19,26.82 v31.5,27.13 | U1.10 43.45,33.5 43.89,33.93 44.6,33.93 v44.91,34.24
MOSI_LV  (via drill 0.41)
  Top 0.203: v21.95,30.07 20.12,28.25 18.67,28.25 X1_NM.7
  Bottom 0.203: IC1.6 28.12,28.07 27.03,29.26 26.11,29.26 25.6,28.75 23.27,28.75 v21.95,30.07 18.66,33.36 18.66,36.31 15.85,39.12 15.85,44.99 U2.3
N$1  (via drill 0.41)
  other vias: 26.62,28.45
N$2
  Bottom 0.203: R2.1 28.55,22.96 | 28.55,22.96 28.75,23.16 28.88,23.88 SJ1.2 | 28.55,22.96 28.55,20.24 T1.3
N$3
  Bottom 0.406: C1.1 13.88,22.07 IC2.4
N$4  (via drill 0.41)
  Top 0.203: LED0.A 73.22,42.5 73.46,42.27 73.46,41.5 v73.47,41.49
  Bottom 0.203: RN4.8 v73.47,41.49
N$5  (via drill 0.41)
  Top 0.203: LED2.A 75.22,17.17 75.29,17.17 75.39,17.27 v75.39,26.72
  Bottom 0.203: v75.39,26.72 74.98,27.13 74.98,33.12 77.42,35.56 77.42,41.35 RN4.5
N$6  (via drill 0.41)
  Top 0.203: v72.24,29.46 72.24,18.9 70.34,17 LED1.A
  Bottom 0.203: v72.24,29.46 72.24,31.29 76.61,35.66 76.61,41.39 RN4.6
N$7  (via drill 0.41)
  Top 0.203: BTN_A.3 BTN_A.4 19.49,2.54 v21.03,2.54
  Bottom 0.203: RN2.5 27.14,5.4 24.28,2.54 v21.03,2.54
N$8
  Bottom 0.406: SD_MISO.1 26.11,40.77 IC3.4
N$9
  Bottom 0.203: 31.6,5.32 RN2.8 RN2.7
N$10
  Bottom 0.203: RN6.6 RN6.5
N$11  (via drill 0.41)
  Top 0.203: BTN_B.3 30.79,2.5 | 30.79,2.5 BTN_B.4 | v30.79,3.05 30.79,2.5
  Bottom 0.203: v30.79,3.05 30.79,3.95 RN2.2
N$12  (via drill 0.41)
  Top 0.203: BTN_C.3 47.85,2.5 | 47.85,2.5 BTN_C.4 | v47.85,3.76 47.85,2.5
  Bottom 0.203: RN6.1 47.51,4.1 v47.85,3.76
N$13
  Bottom 0.203: RN6.2 RN6.3
N$14
  Bottom 0.203: RN6.8 RN6.7
SCLK  (via drill 0.41)
  Top 0.203: v19.71,37.19 7.21,37.19 ICSP.3 | v32.72,35.05 33.02,35.36 43.38,35.36 v43.69,35.05
  Bottom 0.203: v19.71,37.19 19.71,34.95 22.15,32.51 28.14,32.51 28.78,31.88 IC1.3 29.79,31.8 30.48,31.9 30.68,31.9 31.11,32.33 31.11,33.45 v32.72,35.05 | U1.9 42.95,33.91 43.48,34.44 43.48,34.85 v43.69,35.05
SCLK_LV  (via drill 0.41)
  Top 0.203: v15.65,38.22 15.65,38.2 | 15.65,38.2 14.71,39.14 v13.63,39.14 | v19.3,30.28 18.09,29.06 15.64,29.06 X1_NM.6 | 15.65,38.2 22.86,38.2 23.27,37.8 v23.27,37.39
  Bottom 0.203: IC1.2 29.72,33.07 29.67,33.12 28.75,33.12 28.14,33.73 27.43,33.73 27.03,34.14 26.21,34.14 25.81,33.73 23.57,33.73 23.27,34.04 v23.27,37.39 | v13.63,39.14 13.61,39.12 13.61,45.03 U2.5 | v15.65,38.22 18.19,35.68 18.19,33.02 19.3,31.9 v19.3,30.28
SD_CS_LV
  Bottom 0.203: IC1.12 23.9,29.34 23.67,29.46 | 23.67,29.46 23.77,29.36 | 23.67,29.46 19.2,33.93 19.2,36.58 16.97,38.81 16.97,44.47 U2.2
UCAP
  Bottom 0.203: U1.6 41.45,35.18 C7.1
UGND
  Bottom 0.203: 43.69,44.4 43.59,44.5 | U1.5 40.95,36.46 C7.2 41.81,36.83 43.69,38.71 43.69,42.45 L2.1
  Bottom 0.406: J1.P5 40.69,44.96 41.15,44.5 43.59,44.5 43.69,44.6 | 43.69,44.6 45.01,45.92 USB_GND.2 | 43.69,44.6 43.69,44.52 L2.1
USB_D+
  Bottom 0.203: U1.4 40.45,38.04 RN3.7
USB_D-
  Bottom 0.203: U1.3 39.95,38.03 RN3.8
USB_VCC  (via drill 0.41)
  Top 0.203: v44.5,36.88 v38.3,36.88
  Bottom 0.203: v38.3,36.88 38.3,38.41 F1.1 | U1.7 41.95,34.94 42.9,35.89 43.43,35.89 44.42,36.88 v44.5,36.88
  Bottom 0.406: F1.1 36.33,39.65 C8.+ 32.64,40.23 30.79,40.23 30.76,40.26 C9.1 28.96,41.78 28.96,42.67 29.72,43.43 USB_PWR.1
XTAL1
  Bottom 0.203: U1.17 46.66,29.77 R1.1 48.28,28.14 48.87,28.14 49.29,27.72 X1.3 49.3,27.59 C4.1
XTAL2
  Bottom 0.203: U1.16 46.75,30.27 R1.2 47.55,30.86 47.55,30.89 49.28,30.89 | 49.28,30.89 50.19,30.89 51.1,29.97 51.1,29.9 X1.1 | C3.2 49.3,30.91 49.28,30.89
XUSB
  Bottom 0.406: J1.P1 38.05,44.32 F1.2

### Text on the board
bPlace: INTERFACE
